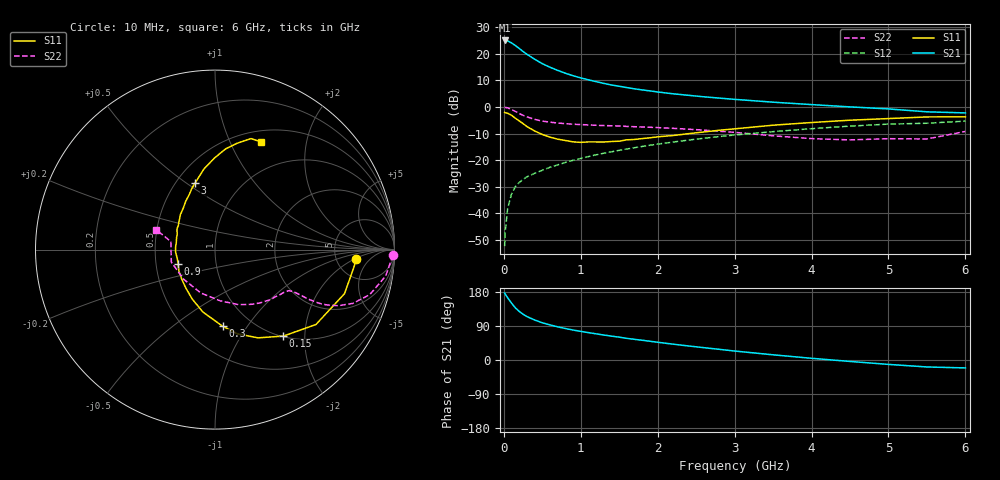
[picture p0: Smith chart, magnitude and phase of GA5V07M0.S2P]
! Infineon Technologies  Discrete & RF Semiconductors
! BF775
! Si NPN RF Bipolar Junction Transistor in SOT23
! VCE = 5 V  IC = 7 mA
! Common Emitter S-Parameters:  May  1996
# GHz  S  MA  R  50
!  f  S11  S21  S12  S22
! GHz  MAG  ANG  MAG  ANG  MAG  ANG  MAG  ANG
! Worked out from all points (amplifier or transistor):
!   36 points, 10 MHz to 6 GHz, reference 50 ohm
!   highest |S21| = 25.1 dB at 10 MHz (marker M1)
!   |S21| within 3 dB of that: start of sweep to 199.9 MHz
!   unconditionally stable (mu >= 1): 715.7 MHz to 3.129 GHz
!   at 250 MHz: K = 0.57, MSG = 24.1 dB, |S12| = -27.3 dB
!   at 1.4 GHz: K = 1.11, MAG = 10.5 dB, |S12| = -16.9 dB
!   at 6 GHz: K = 0.93, MSG = 1.5 dB, |S12| = -5.3 dB
!   S11 on the Smith chart (normalised r, x): 10 MHz: 7.90, -2.13; 150 MHz: 1.01, -1.56; 300 MHz: 0.74, -0.78; 900 MHz: 0.65, -0.11; 3 GHz: 0.62, +0.54; 6 GHz: 0.63, +1.32
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0.01  0.789 -3.7  17.89 176.7  0.0024 90.8  0.9903 -1.7
0.02  0.7791 -7.6  17.86 173.2  0.0048 84.7  0.9828 -3.6
0.05  0.7621 -18.8  17.59 164.0  0.0124 81.4  0.9624 -8.8
0.1  0.7003 -36.6  16.07 150.1  0.023 71.6  0.8982 -16.2
0.15  0.614 -51.7  14.34 137.4  0.0317 66.5  0.8246 -21.3
0.2  0.547 -64.0  12.66 128.2  0.038 63.3  0.7543 -24.5
0.25  0.486 -75.0  11.08 120.8  0.0434 61.2  0.6967 -26.3
0.3  0.4285 -84.4  9.824 114.6  0.0485 60.1  0.6518 -27.3
0.4  0.3539 -101.1  7.937 105.6  0.0564 59.9  0.5849 -28.0
0.5  0.3037 -114.5  6.538 98.2  0.0645 60.1  0.5425 -28.0
0.6  0.2707 -126.4  5.595 92.6  0.0733 60.6  0.5183 -28.1
0.7  0.2481 -138.2  4.892 87.5  0.0815 61.6  0.4995 -28.2
0.9  0.2206 -158.5  3.878 79.1  0.0992 62.0  0.4739 -28.9
1.1  0.2202 -176.4  3.246 72.3  0.1167 62.1  0.459 -30.8
1.3  0.2193 169.3  2.779 65.9  0.1348 61.5  0.4472 -32.9
1.6  0.2412 151.5  2.316 57.1  0.1621 60.0  0.431 -36.9
2.2  0.2903 127.6  1.772 41.8  0.2192 55.7  0.3967 -47.4
3  0.388 106.5  1.393 23.7  0.297 47.8  0.3332 -66.9
3.5  0.4543 97.7  1.232 13.7  0.3438 41.9  0.2868 -84.3
4.5  0.5642 84.0  1.005 -3.8  0.4364 29.2  0.2403 -136.3
5.5  0.6503 72.0  0.811 -18.4  0.4947 14.3  0.25 169.6
6  0.6526 66.8  0.774 -20.9  0.5422 10.1  0.3467 161.3
